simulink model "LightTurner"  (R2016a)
settings: Solver=FixedStepAuto  StartTime=0.0  StopTime=inf  RelTol=1e-3
libraries: miniQ x2

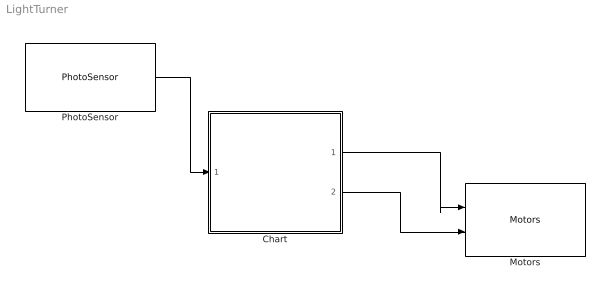
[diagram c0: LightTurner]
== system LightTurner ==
  Chart : Stateflow chart  TreatAsAtomicUnit=on
  Motors : miniQ/Motors  flipLeft=off  flipRight=off
  PhotoSensor : miniQ/PhotoSensor  sampleTime_dd=0.01  debug_dd=off
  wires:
  PhotoSensor/1 -> Chart/1(lite)
  Chart/1(l) -> Motors/1
  Chart/2(r) -> Motors/2

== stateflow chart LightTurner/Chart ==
  state Stop
    entry: l= 0
    r=0
  state Right
    entry: l=200
    r=-200
  state Left
    entry: l=-200
    r=200
  (default) -> Stop
  Right -> Stop : [lite<900]
  Left -> Stop : [lite>30]
  Stop -> Left : [lite<30]
  Stop -> Right : [lite>900]
  data: l output; r output; lite input
